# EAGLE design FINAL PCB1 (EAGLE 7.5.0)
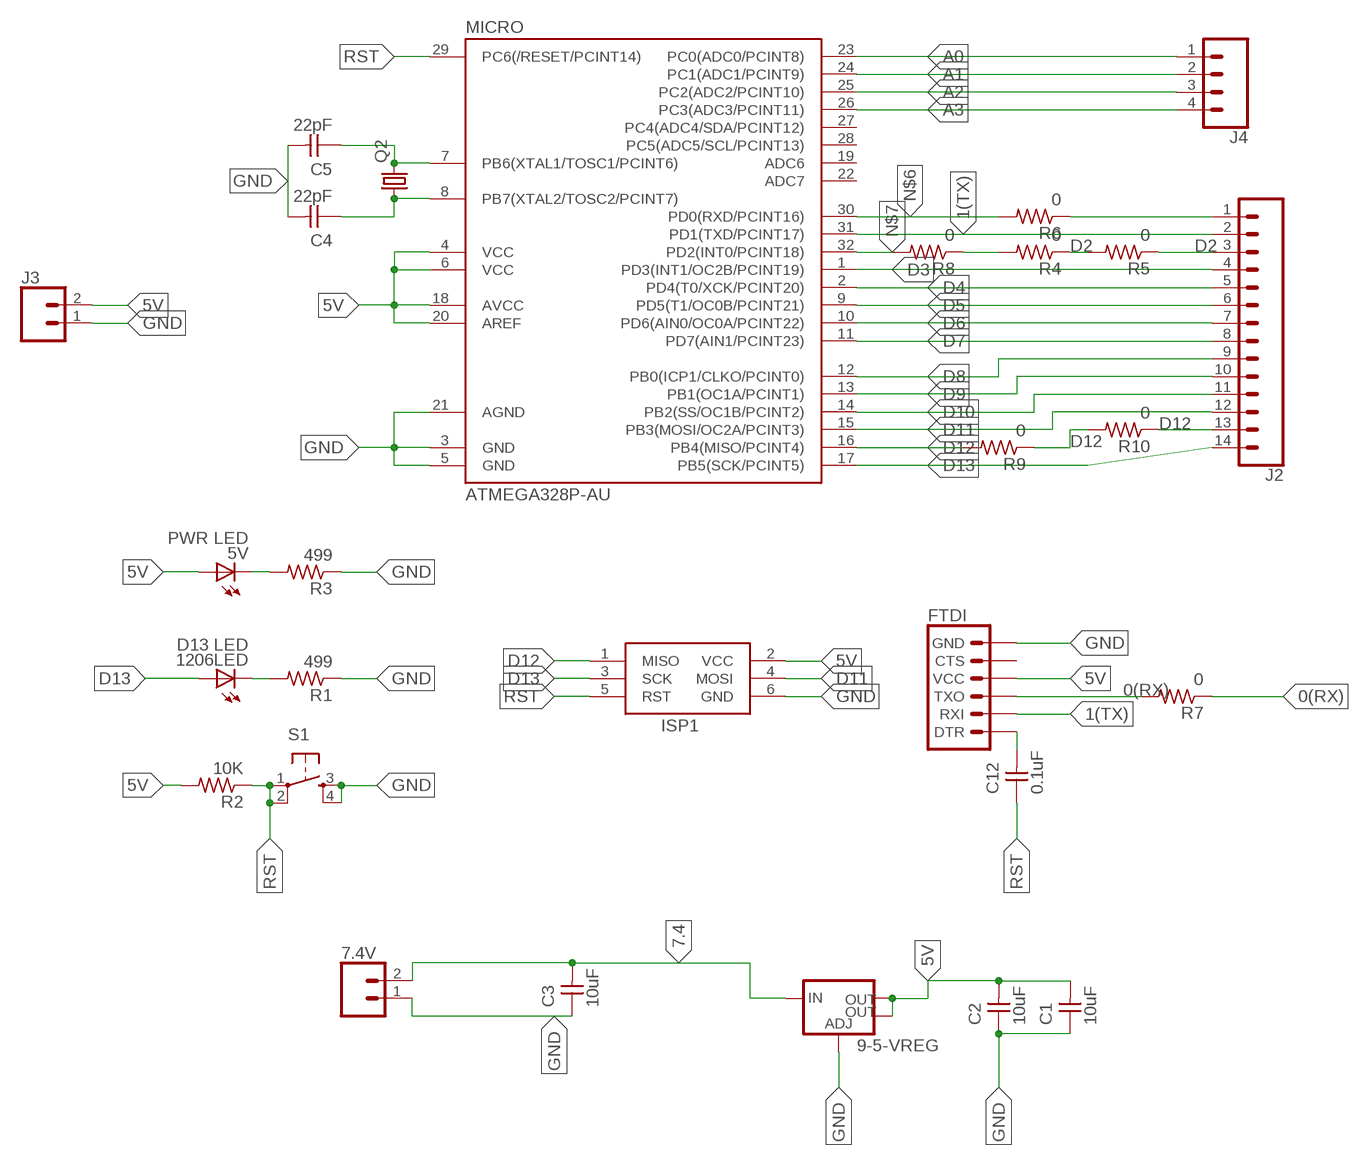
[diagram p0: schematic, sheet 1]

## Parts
5V  PWR LED  LEDFAB1206  [LED1206FAB]
7.4V  CONN_02LOCK  [1X02_LOCK]
9-5-VREG  V_REG_LM1117SOT223  [SOT223]
1206LED  D13 LED  LEDFAB1206  [LED1206FAB]
C1  10uF  CAP-UNPOLARIZEDFAB  [C1206FAB]
C2  10uF  CAP-UNPOLARIZEDFAB  [C1206FAB]
C3  10uF  CAP-UNPOLARIZEDFAB  [C1206FAB]
C4  22pF  CAP-UNPOLARIZEDFAB  [C1206FAB]
C5  22pF  CAP-UNPOLARIZEDFAB  [C1206FAB]
C12  0.1uF  CAP-UNPOLARIZEDFAB  [C1206FAB]
FTDI  6_PIN_SERIAL_TARGET_SILK  [1X06]
ISP1  AVRISP-6  [AVRISP]
J2  CONN_14  [1X14]
J3  CONN_02  [1X02]
J4  CONN_04  [1X04]
MICRO  ATMEGA328P-AU  ATMEGA48/88/168-AU  [TQFP32-08]
Q2  CRYSTALHC49U70  [HC49U70]
R1  499  RES-US1206FAB  [R1206FAB]
R2  10K  RES-US1206FAB  [R1206FAB]
R3  499  RES-US1206FAB  [R1206FAB]
R4  0  RES-US1206FAB  [R1206FAB]
R5  0  RES-US1206FAB  [R1206FAB]
R6  0  RES-US1206FAB  [R1206FAB]
R7  0  RES-US1206FAB  [R1206FAB]
R8  0  RES-US1206FAB  [R1206FAB]
R9  0  RES-US1206FAB  [R1206FAB]
R10  0  RES-US1206FAB  [R1206FAB]
S1  6MM_SWITCH6MM_SWITCH  [6MM_SWITCH]

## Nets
0(RX): FTDI.3(TXO) J2.1 R6.1 R7.1 R7.2
1(TX): FTDI.2(RXI) J2.2 MICRO.31(PD1(TXD/PCINT17))
5V: 5V.1(A) 9-5-VREG.2(OUT) 9-5-VREG.4(OUT) C1.2 C2.2 FTDI.4(VCC) ISP1.2(VCC) J3.2 MICRO.4(VCC) MICRO.6(VCC) MICRO.18(AVCC) MICRO.20(AREF) R2.2
7.4: 7.4V.2 9-5-VREG.3(IN) C3.2
A0: J4.1 MICRO.23(PC0(ADC0/PCINT8))
A1: J4.2 MICRO.24(PC1(ADC1/PCINT9))
A2: J4.3 MICRO.25(PC2(ADC2/PCINT10))
A3: J4.4 MICRO.26(PC3(ADC3/PCINT11))
D2: J2.3 R4.1 R4.2 R5.1 R5.2 R8.1
D3: J2.4 MICRO.1(PD3(INT1/OC2B/PCINT19))
D4: J2.5 MICRO.2(PD4(T0/XCK/PCINT20))
D5: J2.6 MICRO.9(PD5(T1/OC0B/PCINT21))
D6: J2.7 MICRO.10(PD6(AIN0/OC0A/PCINT22))
D7: J2.8 MICRO.11(PD7(AIN1/PCINT23))
D8: J2.9 MICRO.12(PB0(ICP1/CLKO/PCINT0))
D9: J2.10 MICRO.13(PB1(OC1A/PCINT1))
D10: J2.11 MICRO.14(PB2(SS/OC1B/PCINT2))
D11: ISP1.4(MOSI) J2.12 MICRO.15(PB3(MOSI/OC2A/PCINT3))
D12: ISP1.1(MISO) J2.13 MICRO.16(PB4(MISO/PCINT4)) R9.1 R9.2 R10.1 R10.2
D13: 1206LED.1(A) ISP1.3(SCK) J2.14 MICRO.17(PB5(SCK/PCINT5))
GND: 7.4V.1 9-5-VREG.1(ADJ) C1.1 C2.1 C3.1 C4.2 C5.2 FTDI.6(GND) ISP1.6(GND) J3.1 MICRO.3(GND) MICRO.5(GND) MICRO.21(AGND) R1.1 R3.1 S1.3(S) S1.4(S1)
N$1: 1206LED.2(C) R1.2
N$2: 5V.2(C) R3.2
N$3: C5.1 MICRO.7(PB6(XTAL1/TOSC1/PCINT6)) Q2.2
N$4: C4.1 MICRO.8(PB7(XTAL2/TOSC2/PCINT7)) Q2.1
N$6: MICRO.30(PD0(RXD/PCINT16)) R6.2
N$7: MICRO.32(PD2(INT0/PCINT18)) R8.2
N$16: C12.2 FTDI.1(DTR)
RST: C12.1 ISP1.5(RST) MICRO.29(PC6(/RESET/PCINT14)) R2.1 S1.1(P) S1.2(P1)
Unconnected: FTDI.5(CTS) MICRO.19(ADC6) MICRO.22(ADC7) MICRO.27(PC4(ADC4/SDA/PCINT12)) MICRO.28(PC5(ADC5/SCL/PCINT13))

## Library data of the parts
5V 1206LED = fab:LED: LED
7.4V J3 = SparkFun-Connectors:CONN_02: Multi connection point. Often used as Generic Header-pin footprint for 0.1 inch spaced/style header connections
9-5-VREG = fab:V_REG_LM1117: Voltage Regulator LM1117 Standard adjustable voltage regulator but in SMD form. Spark Fun Electronics SKU : COM-00595; PROD_ID: VREG-08170
C1-C5 C12 = fab:CAP-UNPOLARIZED
FTDI = SparkFun-Connectors:6_PIN_SERIAL_TARGET: 6-pin header connection for use with the "FTDI BASIC" pinout - TARGET SIDE. Also known as "Arduino Serial Program Header". It is used to mate with our FTDI Basic serial programmers using the Arduino IDE. Note, this device has "TARGET" in the name. It is intended to be used on a design that contains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
ISP1 = adafruit:AVRISP: AVR ISP HEADER Standard 6 pin header for AVR programming
J2 = SparkFun-Connectors:CONN_14: Multi connection point. Often used as Generic Header-pin footprint for 0.1 inch spaced/style header connections On any of the 0.1 inch spaced packages, you can populate with these: Break Away Headers - Straight (PRT-00116) Break Away Male Headers - Right Angle (PRT-00553) Female Headers (PRT-00115)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
J4 = SparkFun-Connectors:CONN_04: Multi connection point. Often used as Generic Header-pin footprint for 0.1 inch spaced/style header connections On any of the 0.1 inch spaced packages, you can populate with these: Break Away Headers - Straight (PRT-00116) Break Away Male Headers - Right Angle (PRT-00553) Female Headers (PRT-00115)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; PROD_ID: CONN-09696
MICRO = atmega8:ATMEGA48/88/168
Q2 = crystal:CRYSTAL: CRYSTAL; OC_FARNELL: unknown; OC_NEWARK: unknown
R1-R10 = fab:RES-US: Resistor (US Symbol)
S1 = fab:6MM_SWITCH: OMRON SWITCH

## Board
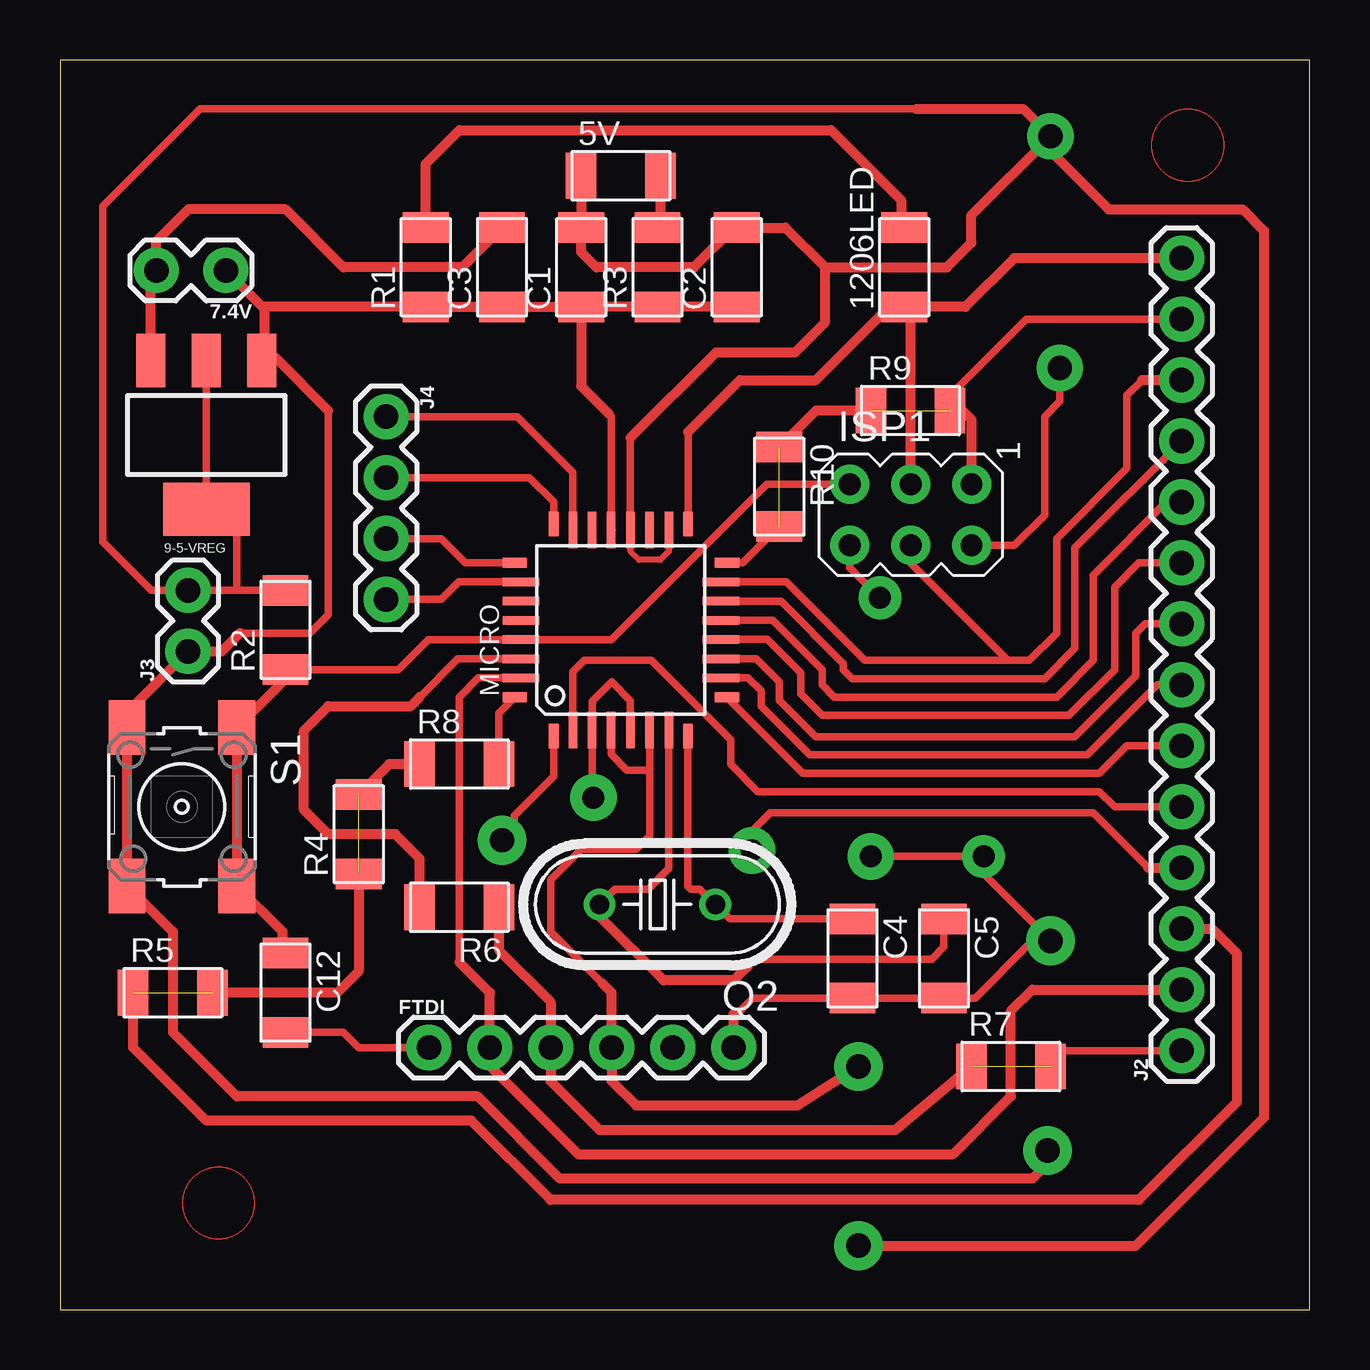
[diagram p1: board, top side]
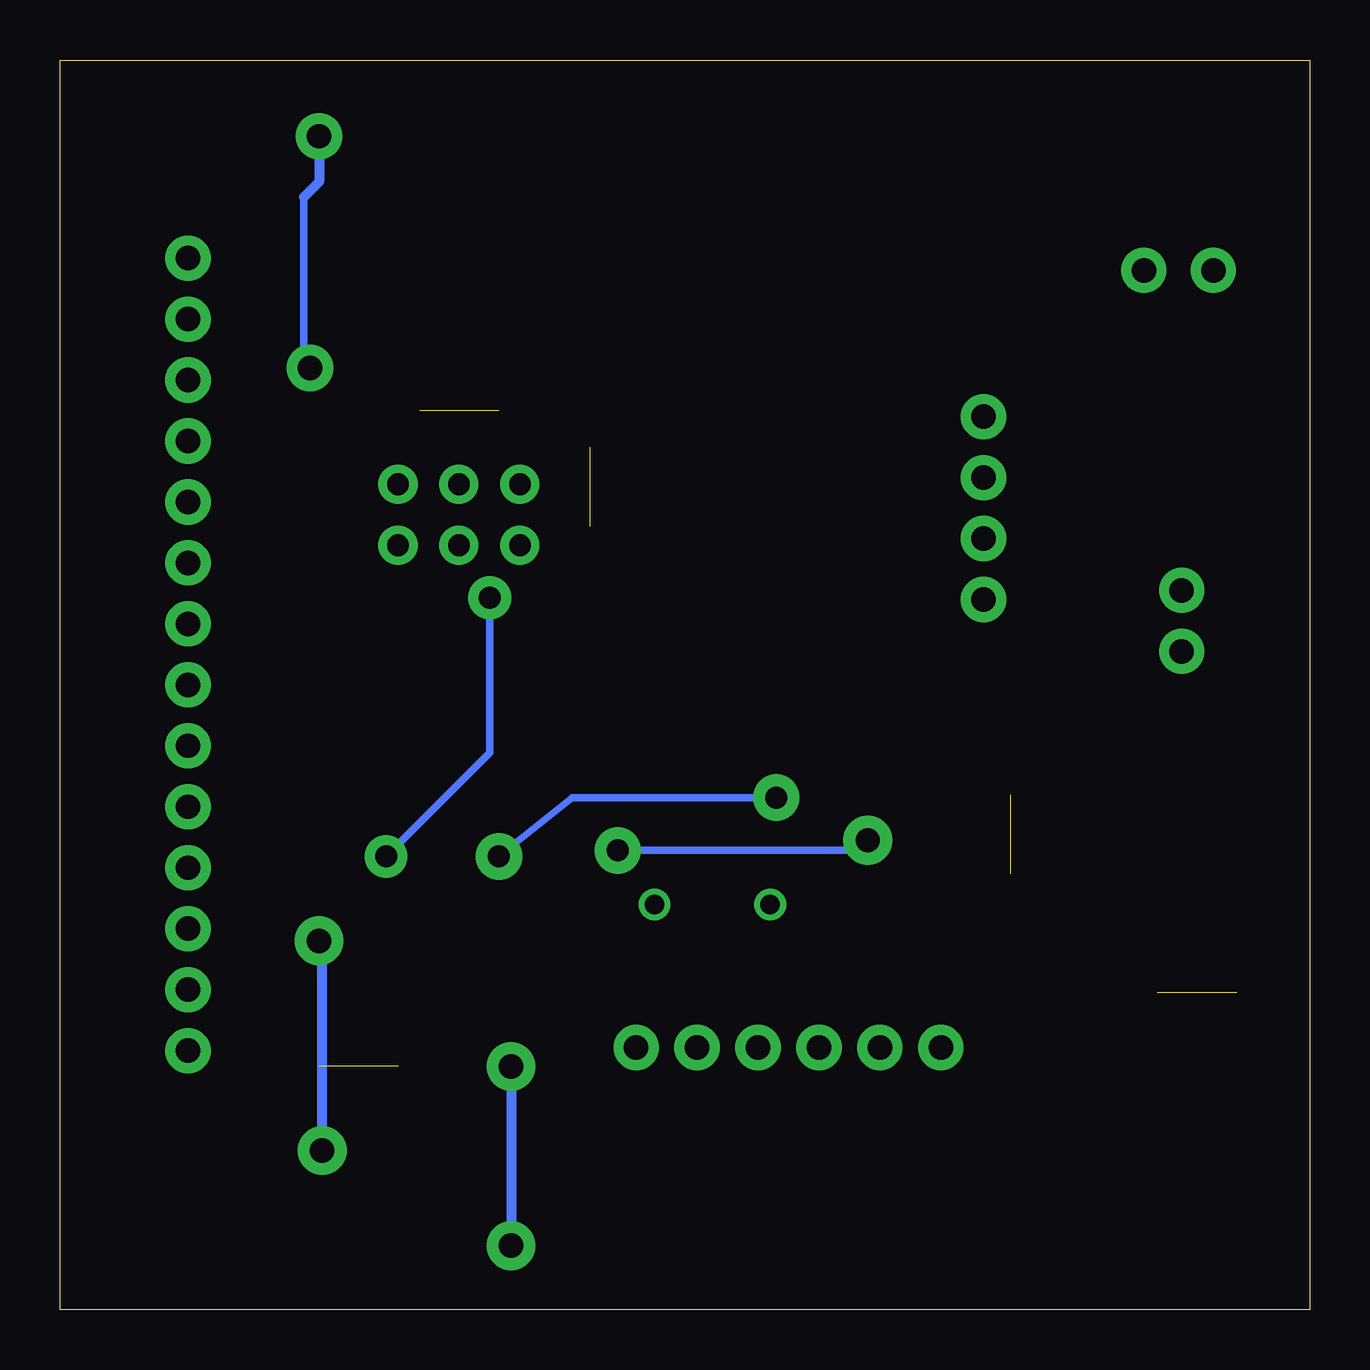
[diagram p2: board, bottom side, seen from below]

Size 52.07 x 52.07 mm. Coordinates in mm from the lower left corner, seen from the top.
Outline: 0,0 52.07,0 52.07,52.07 0,52.07 0,0
Copper layers (1*16): Top 0.035mm / dielectric 1.5mm / Bottom 0.035mm
Design rules "default *": minimum track width 10mil, minimum drill 24mil, track to track 12mil, track to pad 12mil, pad to pad 12mil, via to via 12mil, smd to smd 8mil, copper to edge 40mil, drill to drill 8mil, minimum pad ring 10mil, minimum via ring 8mil, stop-mask expansion 4mil, vias tented up to drill 0mil, thermal gap 10mil

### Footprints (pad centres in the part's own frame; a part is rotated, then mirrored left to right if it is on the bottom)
LED1206FAB = smd 1.27 x 1.905: 1 -1.651,0; 2 1.651,0
1X02_LOCK = drill 1.016 pad 1.88: 1 -0.178,0; 2 2.718,0
SOT223 = smd 1.219 x 2.235: 1 -2.311,-3.099; 2 0,-3.099; 3 2.311,-3.099 | smd 3.6 x 2.2: 4 0,3.099
C1206FAB = smd 1.27 x 1.905: 1 -1.651,0; 2 1.651,0
1X06 = drill 1.016 pad 1.88: 1 0,0; 2 2.54,0; 3 5.08,0; 4 7.62,0; 5 10.16,0; 6 12.7,0
AVRISP = drill 0.9 pad 1.626: 1 -1.27,2.54; 2 1.27,2.54; 3 -1.27,0; 4 1.27,0; 5 -1.27,-2.54; 6 1.27,-2.54
1X14 = drill 1.016 pad 1.88: 1 0,0; 2 2.54,0; 3 5.08,0; 4 7.62,0; 5 10.16,0; 6 12.7,0; 7 15.24,0; 8 17.78,0; 9 20.32,0; 10 22.86,0; 11 25.4,0; 12 27.94,0; 13 30.48,0; 14 33.02,0
1X02 = drill 1.016 pad 1.88: 1 0,0; 2 2.54,0
1X04 = drill 1.016 pad 1.88: 1 0,0; 2 2.54,0; 3 5.08,0; 4 7.62,0
TQFP32-08 = smd 1.016 x 0.406: 1 -4.42,2.8; 8 -4.42,-2.8; 17 4.42,-2.8; 24 4.42,2.8 | smd 1.524 x 0.356: 2 -4.166,2; 3 -4.166,1.2; 4 -4.166,0.4; 5 -4.166,-0.4; 6 -4.166,-1.2; 7 -4.166,-2; 18 4.166,-2; 19 4.166,-1.2; 20 4.166,-0.4; 21 4.166,0.4; 22 4.166,1.2; 23 4.166,2 | smd 0.406 x 1.016: 9 -2.8,-4.42; 16 2.8,-4.42; 25 2.8,4.42; 32 -2.8,4.42 | smd 0.356 x 1.524: 10 -2,-4.166; 11 -1.2,-4.166; 12 -0.4,-4.166; 13 0.4,-4.166; 14 1.2,-4.166; 15 2,-4.166; 26 2,4.166; 27 1.2,4.166; 28 0.4,4.166; 29 -0.4,4.166; 30 -1.2,4.166; 31 -2,4.166
HC49U70 = drill 0.813: 1 -2.413,0; 2 2.413,0
R1206FAB = smd 1.27 x 1.905: 1 -1.651,0; 2 1.651,0
6MM_SWITCH = smd 2.286 x 1.524: 1 -3.302,2.286; 2 3.302,2.286; 3 -3.302,-2.286; 4 3.302,-2.286

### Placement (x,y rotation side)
5V  23.37,47.24 0 top
7.4V  6.73,43.31 180 top
9-5-VREG  6.1,36.45 180 top
1206LED  35.18,43.43 90 top
C1  21.72,43.43 90 top
C2  28.19,43.43 90 top
C3  18.41,43.43 90 top
C4  33.02,14.63 270 top
C5  36.83,14.63 270 top
C12  9.4,13.21 270 top
FTDI  15.37,10.92 0 top
ISP1  35.45,33.12 270 top
J2  46.74,10.79 90 top
J3  5.33,27.43 90 top
J4  13.59,37.21 270 top
MICRO  23.37,28.32 90 top
Q2  24.89,16.89 180 top
R1  15.24,43.43 90 top
R2  9.4,28.32 90 top
R3  24.89,43.43 90 top
R4  12.45,19.81 90 top
R5  4.7,13.21 0 top
R6  16.64,16.76 180 top
R7  39.62,10.13 0 top
R8  16.64,22.73 0 top
R9  35.43,37.47 0 top
R10  29.97,34.29 270 top
S1  5.08,20.95 270 top

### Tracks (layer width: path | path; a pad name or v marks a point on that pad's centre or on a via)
0(RX)  (1 unrouted)
  Top 0.305: J2.1 41.4,10.79 R7.2
  Top 0.406: R6.1 18.29,14.99 20.45,12.83 FTDI.3 20.45,9.53 22.48,7.49 34.8,7.49 R7.1
1(TX)
  Top 0.305: 16.64,14.48 16.64,25.53 17.43,26.32 MICRO.31
  Top 0.406: 16.64,14.48 17.91,13.21 FTDI.2 17.91,10.16 21.59,6.48 37.21,6.48 39.62,8.89 39.62,12.45 40.51,13.34 J2.2
5V  (via drill 1.02 pad 1.93, 1.02 pad 2.03)
  Top 0.254: 6.2,39.42 9-5-VREG.2 6.33,39.4 | 6.2,33.55 6.12,33.39 9-5-VREG.4 | 6.33,33.53 9-5-VREG.4 | 9.17,30.18 R2.2 | 6.04,33.25 9-5-VREG.4 | MICRO.18 25.37,31.59 25.02,31.24 24.13,31.24 23.77,31.6 MICRO.20
  Top 0.305: J3.2 R2.2 | J3.2 7.37,29.97 7.37,33.39 6.12,33.39 6.1,33.39 9-5-VREG.2 | J3.2 3.81,29.97 1.78,32 1.78,45.97 5.84,50.04 35.69,50.04 | MICRO.20 23.77,36.32 | v41.66,39.24 41.66,37.85 41.02,37.21 41.02,33.11 39.77,31.85 ISP1.2 | 22.61,13.59 20.45,15.75 20.45,17.91 21.72,19.18 24,19.18 24.57,19.74 24.57,22.48 | MICRO.6 24.57,22.48 | MICRO.4 22.97,23.13 23.62,22.48 24.57,22.48
  Top 0.406: 35.69,50.04 40.13,50.04 v41.27,48.9 | 31.88,43.43 36.96,43.43 37.97,44.45 37.97,45.59 v41.27,48.9 | 31.88,43.43 30.23,45.09 C2.2 28.07,45.09 26.42,43.43 22.35,43.43 21.72,44.07 C1.2 5V.1 | 31.88,43.43 31.88,41.15 30.61,39.88 27.32,39.88 23.77,36.32 | v33.27,10.13 30.73,8.51 24,8.51 22.99,9.53 FTDI.4 22.99,13.21 22.61,13.59 | v33.27,2.67 44.83,2.67 50.16,8 50.16,44.96 49.28,45.85 43.69,45.85 41.27,48.26 v41.27,48.9
  Bottom 0.305: v41.66,39.24 41.91,39.5 41.91,46.35
  Bottom 0.406: v41.27,48.9 41.27,46.99 41.91,46.35 | v33.27,10.13 v33.27,2.67
7.4
  Top 0.406: 9-5-VREG.3 3.79,43.08 7.4V.2 4.01,44.53 5.33,45.85 9.4,45.85 11.81,43.43 16.76,43.43 C3.2
A0
  Top 0.254: 21.31,32.54 MICRO.23
  Top 0.305: J4.1 19.05,37.21 21.37,34.89 MICRO.23
A1
  Top 0.254: 20.52,32.77 MICRO.24
  Top 0.305: MICRO.24 20.57,33.66 19.55,34.67 J4.2
A2
  Top 0.305: MICRO.25 16.89,31.12 15.88,32.13 J4.3
A3
  Top 0.305: J4.4 15.88,29.59 16.61,30.32 MICRO.26
D2  (2 unrouted)
  Top 0.406: R4.1 12.45,14.1 11.56,13.21 R5.2 | R8.1 13.72,22.73 R4.2 | R5.1 3.05,10.92 6.1,7.87 17.14,7.87 20.45,4.57 44.96,4.57 49.02,8.64 49.02,14.86 48.01,15.88 J2.3
D3  (via drill 0.91 pad 1.93, 1.02 pad 2.03)
  Top 0.305: MICRO.1 20.57,22.22 18.92,20.57 18.92,20.07 v18.41,19.56 | v28.83,19.14 28.83,19.94 29.59,20.7 43.05,20.7 45.34,18.41
  Top 0.406: 45.34,18.41 J2.4
  Bottom 0.305: v28.83,19.14 18.84,19.14 v18.41,19.56
D4
  Top 0.305: MICRO.2 21.37,26.57 21.84,27.05 24.65,27.05 27.69,24.01 27.94,23.76 27.94,22.73 29.08,21.59 43.31,21.59 43.94,20.95 J2.5
D5
  Top 0.254: 27.79,25.5 MICRO.9
  Top 0.305: MICRO.9 30.96,22.35 43.31,22.35 44.45,23.5 J2.6
D6
  Top 0.254: 27.79,26.34 MICRO.10
  Top 0.305: 27.79,26.34 28.65,26.34 29.21,25.78 29.21,25.15 31.24,23.11 42.8,23.11 45.72,26.04 J2.7
D7
  Top 0.305: MICRO.11 29.01,27.12 29.97,26.16 29.97,25.4 31.5,23.88 42.29,23.88 44.83,26.42 44.83,28.19 45.21,28.57 J2.8
D8
  Top 0.305: J2.9 44.96,31.11 43.94,30.1 43.94,26.67 42.04,24.77 31.75,24.77 30.86,25.65 30.86,26.54 29.46,27.94 27.55,27.94 MICRO.12
D9
  Top 0.305: MICRO.13 29.7,28.72 31.75,26.67 31.75,26.04 32.26,25.53 41.53,25.53 43.05,27.05 43.05,30.61 46.1,33.66 J2.10
D10
  Top 0.305: MICRO.14 30.04,29.52 32.64,26.92 32.64,26.67 33.02,26.29 41.02,26.29 42.29,27.56 42.29,31.75 J2.11
D11
  Top 0.305: MICRO.15 30.26,30.32 33.53,27.05 39.5,27.05 | 39.5,27.05 40.39,27.05 41.53,28.19 41.53,32.13 44.45,35.05 44.45,38.1 45.09,38.73 | ISP1.4 35.45,31.1 39.5,27.05
  Top 0.406: J2.12 45.09,38.73
D12  (2 unrouted)
  Top 0.254: 28.02,31.14 MICRO.16
  Top 0.305: J2.13 40.26,41.27 37.08,38.1 37.08,37.97 R9.2 37.1,37.07 | MICRO.16 28.45,31.12 R10.2
  Top 0.406: R9.1 31.5,37.47 R10.1 | ISP1.1 37.99,37.07 37.08,37.97
D13
  Top 0.254: 26.11,32.77 MICRO.17
  Top 0.305: MICRO.17 26.17,36.58
  Top 0.406: J2.14 39.75,43.81 37.72,41.78 1206LED.1 | 1206LED.1 35.05,41.91 34.67,41.91 31.5,38.73 28.33,38.73 26.17,36.58 | ISP1.3 35.45,41.52 1206LED.1
GND  (via drill 0.91 pad 1.78, 0.91 pad 1.93, 1.02 pad 2.03)
  Top 0.254: 8.53,39.73 9-5-VREG.1 8.56,39.67 | 22.99,32.54 MICRO.21 | 22.99,32.26 MICRO.21 | MICRO.21 23.04,32.49
  Top 0.305: 9-5-VREG.1 8.41,39.62 | 22.86,37.34 22.97,37.23 MICRO.21 | 7.49,28.19 10.41,28.19 11.18,28.96 11.18,37.47 | v22.23,21.34 22.17,21.39 MICRO.3 22.17,25.34 22.99,26.16 23.77,25.38 MICRO.5 | v33.78,18.89 v38.48,18.89 38.48,18.16 v41.27,15.37 41.15,15.24 40.39,15.24 38.13,12.98 C5.2 C4.2 28.86,12.98 28.07,12.19 | ISP1.6 32.91,30.92 v34.16,29.67
  Top 0.406: 7.49,28.19 6.73,27.43 J3.1 2.79,24.89 S1.3 S1.4 4.7,15.75 4.7,11.56 7.37,8.89 17.4,8.89 20.83,5.46 40.51,5.46 41.15,6.1 v41.15,6.63 | FTDI.6 28.07,12.19 28.07,12.32 | C1.1 C3.1 R1.1 8.51,41.78 | C2.1 R3.1 C1.1 | C1.1 21.72,38.48 22.86,37.34 | 8.51,41.78 8.43,41.78 7.4V.1 | 8.53,39.73 8.53,41.76 8.51,41.78 | 8.56,39.67 8.97,39.67 11.18,37.47
  Bottom 0.305: v22.23,21.34 30.73,21.34 v33.78,18.89 | v34.16,29.67 34.16,23.2 v38.48,18.89
  Bottom 0.406: v41.15,6.63 41.15,15.24 v41.27,15.37
N$1
  Top 0.406: R1.2 15.24,47.75 16.64,49.15 32.13,49.15 35.05,46.23 35.05,45.21 1206LED.2
N$2
  Top 0.406: 5V.2 25.02,45.21 R3.2
N$3
  Top 0.305: MICRO.7 25.37,18.38 24.51,17.53 23.12,17.53 Q2.2 | C5.1 36.83,15.11 36.32,14.61 28.96,14.61 28.64,14.29
  Top 0.406: 28.64,14.29 28.07,13.72 25.15,13.72 22.48,16.38 Q2.2
N$4
  Top 0.254: 26.11,23.82 MICRO.8
  Top 0.305: MICRO.8 26.16,17.65 26.29,17.53 26.66,17.53 Q2.1 27.9,16.29 C4.1
N$6
  Top 0.305: MICRO.30 16.58,27.12 14.99,25.53
  Top 0.406: R6.2 14.99,18.8 13.97,19.81 11.18,19.81 10.16,20.83 10.16,24.13 11.18,25.15 14.61,25.15 14.99,25.53
N$7
  Top 0.254: 19.13,25.5 MICRO.32
  Top 0.305: MICRO.32 18.29,24.86 R8.2
N$16
  Top 0.305: C12.2 11.81,11.56 12.45,10.92 FTDI.1
RST
  Top 0.254: 9.37,14.63 C12.1 9.45,14.91 | 9.45,26.54 R2.1
  Top 0.305: C12.1 9.27,14.99 | ISP1.5 29.44,34.39 22.97,27.92 MICRO.29 15.35,27.92 14.1,26.67 R2.1
  Top 0.406: 9.45,26.54 9.45,26.34 S1.1 S1.2 9.27,15.75 9.27,14.99
(copper drawn outside any net)
  shapes: Top circle x2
